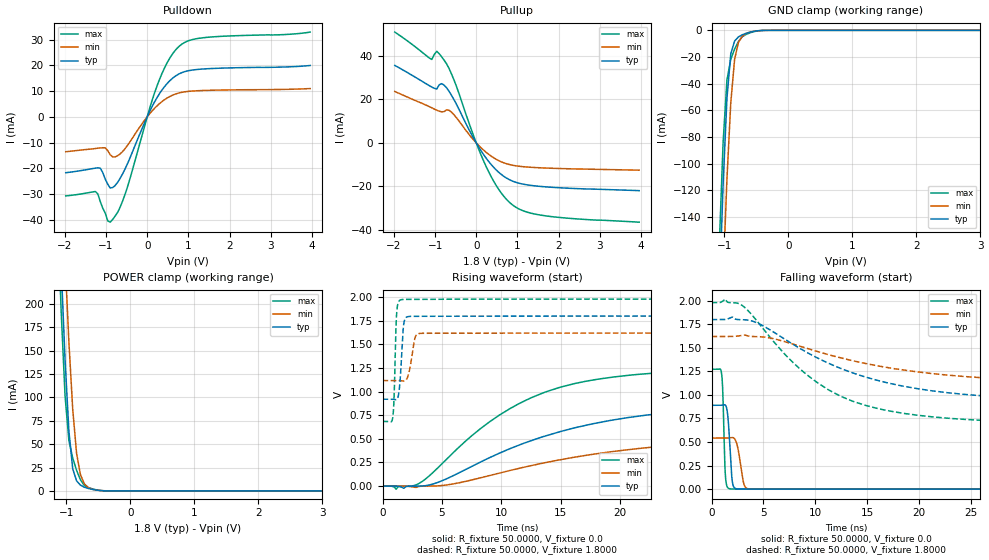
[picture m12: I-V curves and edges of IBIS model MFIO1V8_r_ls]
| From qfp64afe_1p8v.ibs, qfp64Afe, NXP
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[Model] MFIO1V8_r_ls
|   Model MFIO1V8_r_ls
| This model was characterised for following simulation conditions:
| External (pad) voltage:
|   - Typ: 1.8V,   - Min: 1.62V,   - Max: 1.98V
| Library cells for typ/min/max conditions are connected as defined below:
|  IO - External Pad
|  A - Core Input
|  EN - Output Buffer Enable
|  BOOST - vdde
|  EHS - gnd
|  ENZI - vdd
|  EPD - vdd
|  EPUN - gnd
|  ZI - NC
|  ZIF - NC
|  gnd - gnd
|  gnde - gnde
|  vdd - vdd
|  vdde - vdde
| All other pins connected to ground
Model_type I/O
Polarity   Non-Inverting
Enable   Active-Low
Vinl =   0.5400V
Vinh =   1.2600V
Vmeas =  0.9000V
Cref =   0.0F
Rref =   100.0000
Vref =   0.0V
C_comp   1.5958pF   1.5126pF   1.6704pF
|C_comp_pullup   0.7898pF   0.8219pF   0.7460pF
|C_comp_pulldown   0.5931pF   0.6315pF   0.5575pF
[Model Spec]
| variable   typ   min   max
Vinh   0.5400V   0.4860V   0.5940V
Vinl   1.2600V   1.1340V   1.3860V
Vmeas   0.9000V   0.8100V   0.9900V
[Temperature Range]   25.0000   0.1250k   -40.0000
[Voltage Range]   1.8000V   1.6200V   1.9800V
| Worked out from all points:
|   slope of the pulldown table from 0 to 0.27 V, typ, clamps not added: 32.6 ohm
|   slope of the pullup table from 0 to 0.27 V, typ, clamps not added: 34.8 ohm
|   GND clamp passes 1 mA (typ) near -0.56 V on its own axis
|   POWER clamp passes 1 mA (typ) near -0.54 V on its own axis
|   rising waveform, R_fixture 50.0000, V_fixture 0.0: 20-80 % time 13ns typ, 15.7ns min, 9.09ns max; typ from 0 V to 0.89 V
|   rising waveform, R_fixture 50.0000, V_fixture 1.8000: 20-80 % time 250ps typ, 393ps min, 168ps max; typ from 0.92 V to 1.8 V
|   falling waveform, R_fixture 50.0000, V_fixture 0.0: 20-80 % time 296ps typ, 476ps min, 196ps max; typ from 0.89 V to 0 V
|   falling waveform, R_fixture 50.0000, V_fixture 1.8000: 20-80 % time 11.7ns typ, 13.6ns min, 8.54ns max; typ from 1.8 V to 0.92 V
[Pulldown]
|Voltage   I(typ)   I(min)   I(max)
-1.98V    -21.74mA   -13.58mA   -30.76mA
-1.26V    -19.96mA   -12.33mA   -29.04mA
-1.14V    -19.96mA   -12.1mA    -33mA
-960mV    -26.19mA   -13.15mA   -40.44mA
-840mV    -27.51mA   -15.58mA   -39.92mA
-540mV    -20.34mA   -12.41mA   -30.2mA
60mV      2.086mA    1.197mA    3.341mA
300mV     9.043mA    5.145mA    14.58mA
540mV     13.88mA    7.813mA    22.59mA
840mV     17.16mA    9.517mA    28.23mA
1.44V     18.67mA    10.27mA    30.87mA
3.96V     19.95mA    10.98mA    32.93mA
[Pullup]
|Voltage   I(typ)   I(min)   I(max)
-1.98V    35.7mA     23.68mA    51.03mA
-1.08V    25.71mA    16.17mA    38.42mA
-960mV    24.81mA    15.04mA    42.18mA
-840mV    27.29mA    14.27mA    39.65mA
-720mV    25.36mA    15.21mA    36.42mA
-540mV    19.88mA    12.94mA    28.95mA
-60mV     2.001mA    1.263mA    3.041mA
240mV     -7.02mA    -4.333mA   -10.88mA
600mV     -14.41mA   -8.644mA   -22.88mA
900mV     -17.74mA   -10.36mA   -28.83mA
1.74V     -20.33mA   -11.62mA   -33.75mA
3.96V     -22mA      -12.58mA   -36.53mA
[GND_clamp]
|Voltage   I(typ)   I(min)   I(max)
-1.98V    -1.781A    -1.801A    -1.77A
-1.08V    -200.1mA   -270.2mA   -162.2mA
-1.02V    -116mA     -186.2mA   -84.49mA
-960mV    -51.26mA   -111.8mA   -37.36mA
-900mV    -17.65mA   -54.44mA   -21.7mA
-840mV    -8.02mA    -21.7mA    -14.08mA
-780mV    -4.924mA   -8.964mA   -8.313mA
-720mV    -3.338mA   -4.442mA   -4.753mA
-600mV    -1.403mA   -1.338mA   -1.896mA
-480mV    -330.4uA   -347.3uA   -423.3uA
-360mV    -26.82uA   -39.45uA   -30.02uA
3.96V     0A         0A         0A
[POWER_clamp]
|Voltage   I(typ)   I(min)   I(max)
-1.98V    2.119A     2.147A     2.105A
-1.14V    349.2mA    450mA      300.6mA
-1.08V    239.1mA    345.9mA    191.2mA
-1.02V    140.4mA    247.8mA    101.7mA
-960mV    64.08mA    159.3mA    53.89mA
-900mV    23.59mA    87.23mA    35.11mA
-840mV    10.79mA    40.2mA     22.07mA
-780mV    6.218mA    17.5mA     11.92mA
-720mV    4.013mA    7.752mA    6.009mA
-600mV    1.739mA    1.846mA    2.368mA
-360mV    67.5uA     96.07uA    73.34uA
3.96V     0A         0A         0A
[Ramp]
| variable   typ   min   max
dV/dt_r  0.5338/12.9743n   0.3251/15.7284n   0.7629/9.0947n
dV/dt_f  0.5279/11.7427n   0.3013/13.6135n   0.7770/8.5385n
R_load = 50.0000
[Rising Waveform]
R_fixture= 50.0000
V_fixture= 0.0
V_fixture_min= 0.0
V_fixture_max= 0.0
|time   V(typ)   V(min)   V(max)
0s        1.134nV    103.8nV    53.92pV
1.144ns   -56.91uV   19.3uV     -32.56mV
3.258ns   111.2uV    -1.514mV   41.66mV
8.165ns   249.7mV    84.73mV    600.6mV
12.51ns   480.2mV    216.6mV    934.6mV
16.16ns   616.2mV    305.8mV    1.085V
20.26ns   716.9mV    378.9mV    1.167V
27.38ns   811mV      458mV      1.227V
39.28ns   866.2mV    514.3mV    1.26V
100ns     889.6mV    541.8mV    1.272V
[Rising Waveform]
R_fixture= 50.0000
V_fixture= 1.8000
V_fixture_min= 1.6200
V_fixture_max= 1.9800
|time   V(typ)   V(min)   V(max)
0s        919.5mV    1.117V     684.3mV
849ps     919.7mV    1.117V     717.8mV
972.5ps   917.7mV    1.117V     942.9mV
1.194ns   916.1mV    1.117V     1.84V
1.419ns   1.035V     1.116V     1.963V
1.651ns   1.492V     1.113V     1.974V
1.929ns   1.778V     1.117V     1.976V
2.744ns   1.797V     1.573V     1.976V
3.297ns   1.797V     1.617V     1.976V
100ns     1.799V     1.619V     1.979V
[Falling Waveform]
R_fixture= 50.0000
V_fixture= 0.0
V_fixture_min= 0.0
V_fixture_max= 0.0
|time   V(typ)   V(min)   V(max)
0s        889.7mV    541.9mV    1.272V
955.9ps   889.9mV    542mV      1.234V
1.082ns   892mV      541.9mV    1.031V
1.349ns   889.8mV    541.7mV    122.2mV
1.585ns   755.1mV    542.8mV    12.87mV
1.821ns   349.4mV    546mV      2.828mV
2.138ns   23.91mV    543.4mV    1.241mV
3.123ns   891.4uV    53.07mV    1.391mV
3.724ns   1.032mV    1.847mV    1.106mV
100ns     20.55nV    161.7nV    7.273nV
[Falling Waveform]
R_fixture= 50.0000
V_fixture= 1.8000
V_fixture_min= 1.6200
V_fixture_max= 1.9800
|time   V(typ)   V(min)   V(max)
0s        1.799V     1.619V     1.979V
1.309ns   1.8V       1.619V     2.017V
3.074ns   1.798V     1.634V     1.94V
4.724ns   1.747V     1.617V     1.737V
7.571ns   1.556V     1.549V     1.375V
11.22ns   1.339V     1.429V     1.058V
14.75ns   1.193V     1.336V     891.9mV
19.93ns   1.065V     1.243V     783.5mV
39.6ns    936.5mV    1.132V     693.8mV
100ns     919.5mV    1.117V     684.3mV
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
